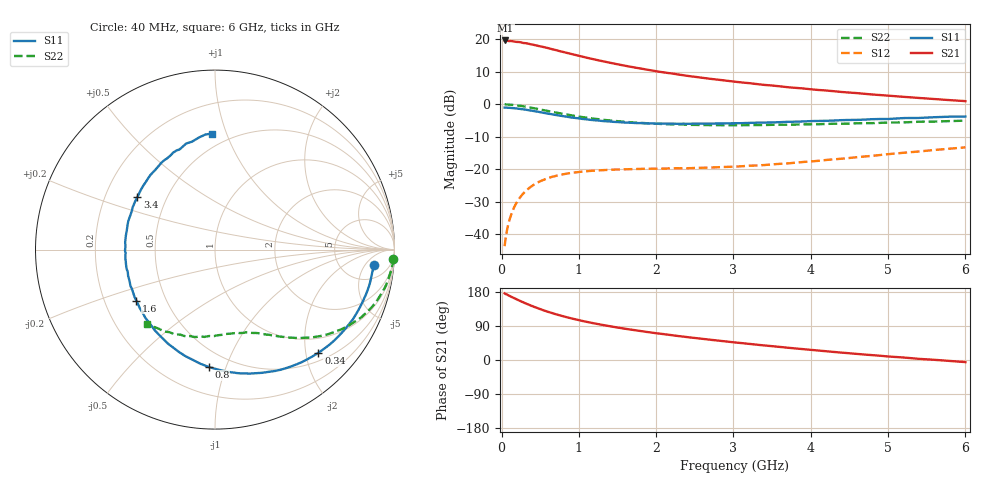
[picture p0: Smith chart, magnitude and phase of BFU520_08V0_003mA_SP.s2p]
! Filename:  P:\Prog\Test\Noise\ATS_data\Testdata_Net\03 Spar\BFU520_APG2013_37_A05_08p0V_003mA_SP_CM01_D.s2p
! Date/Time: Fri 26/Apr/2013 13:00:09
! BFU520_APG2013_37_A05_08p0V_1to20mA_SP_CM01_Bias3_R.s2p
! MDIF S-parameter v. bias file
! BFU520_APG2013_37_A05_08p0V_1to20mA_SP_CM01
! Date/time Tue Apr 23 17:06:44 2013
! VAR V_out= 8.0000
! VAR I_out= 3.0000
! VAR V_in= 0.8124
! VAR I_in= 0.0325
! Device data file deembeded for feedlines and parallel
! Original file: \03 Spar\BFU520_APG2013_37_A05_08p0V_003mA_SP_CM01_R.s2p
! Feed-files: PR047V01_250413_Feed1.s2p, PR047V01_250413_Feed2.s2p
! Parallel-file: PR047V01_250413_Par.s2p
# MHz S MA R 50
!  Freq-MHz  S11-mag  S11-arg  S21-mag  S21-arg  S12-mag  S12-arg  S22-mag  S22-arg
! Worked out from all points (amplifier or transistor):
!   98 points, 40 MHz to 6 GHz, reference 50 ohm
!   highest |S21| = 19.7 dB at 50 MHz (marker M1)
!   |S21| within 3 dB of that: start of sweep to 707 MHz
!   unconditionally stable (mu >= 1): 2.716 GHz to 4.69 GHz
!   at 300 MHz: K = 0.14, MSG = 22.9 dB, |S12| = -27.1 dB
!   at 1.6 GHz: K = 0.65, MSG = 16.0 dB, |S12| = -20.0 dB
!   at 6 GHz: K = 0.83, MSG = 7.1 dB, |S12| = -13.3 dB
!   S11 on the Smith chart (normalised r, x): 40 MHz: 10, -8; 340 MHz: 0.66, -2.25; 800 MHz: 0.38, -0.87; 1.6 GHz: 0.34, -0.26; 3.4 GHz: 0.34, +0.27; 6 GHz: 0.40, +0.89
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40  0.8887 -5.5  9.597 175.8  0.006496 85.9  0.9945 -2.9
50  0.8875 -6.9  9.62 174.1  0.008085 85.4  0.9938 -3.6
60  0.8855 -8.0  9.486 173.6  0.00975 85.1  0.9936 -4.5
70  0.8844 -9.4  9.506 172.8  0.01132 84.3  0.9913 -5.2
120  0.8777 -16.4  9.449 167.5  0.01916 80.3  0.982 -8.9
240  0.8469 -32.5  9.047 155.9  0.03667 71.3  0.9468 -17.4
340  0.8138 -45.0  8.607 147.0  0.04911 64.6  0.9048 -23.7
440  0.7773 -56.9  8.116 138.9  0.05965 58.6  0.8599 -29.2
550  0.7343 -69.2  7.586 130.6  0.06879 52.9  0.8082 -34.6
700  0.6843 -84.1  6.846 120.9  0.07846 46.7  0.7463 -40.5
800  0.6549 -93.2  6.385 115.3  0.08337 43.4  0.7086 -43.8
900  0.626 -101.6  5.967 110.0  0.08739 40.4  0.6769 -46.8
1050  0.5934 -113.1  5.402 102.9  0.09155 36.9  0.633 -50.7
1300  0.5527 -129.8  4.629 92.8  0.09636 32.8  0.5797 -55.8
1600  0.5217 -147.1  3.918 82.4  0.09946 29.8  0.5356 -61.1
2050  0.5038 -167.6  3.158 69.5  0.1016 28.4  0.4977 -68.2
2500  0.5024 175.1  2.651 58.1  0.1043 29.5  0.4809 -75.0
3100  0.511 155.0  2.172 44.7  0.1106 33.1  0.4756 -84.2
3400  0.5221 145.9  1.987 38.4  0.1156 35.0  0.4785 -89.1
4100  0.5527 128.5  1.659 24.9  0.1344 38.9  0.4917 -100.3
5200  0.6123 105.2  1.301 6.6  0.1786 39.5  0.525 -118.7
6000  0.6462 91.5  1.117 -5.5  0.2168 35.9  0.5582 -132.4
